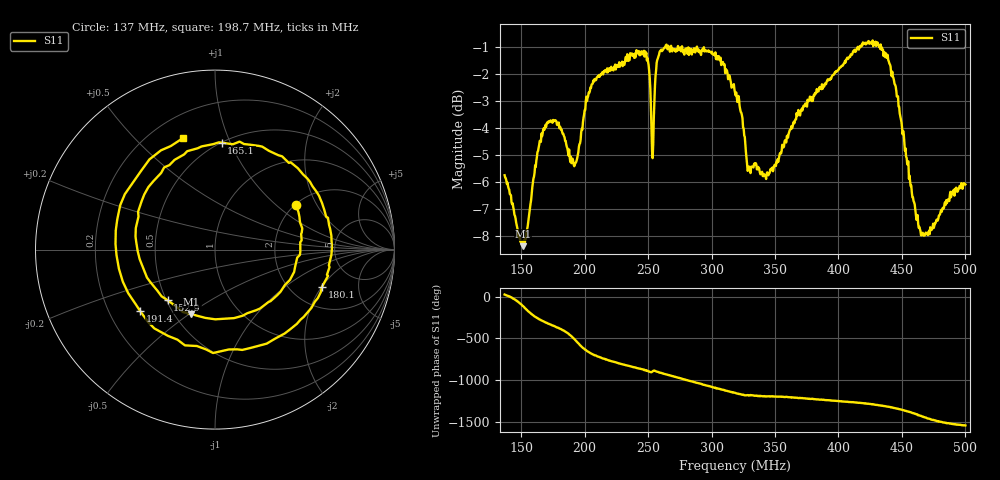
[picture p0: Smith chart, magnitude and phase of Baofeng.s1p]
#  HZ  S  RI  R  50.0
! Rohde & Schwarz ZVL
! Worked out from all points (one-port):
!   801 points, 137 MHz to 500 MHz, reference 50 ohm
!   lowest |S11| = -8.4 dB at 151.5 MHz (marker M1), VSWR 2.23, Z = 30.3 - j25.4 ohm
!   |S11| at or under -10 dB: nowhere
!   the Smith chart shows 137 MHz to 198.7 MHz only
!   S11 on the Smith chart (normalised r, x): 137 MHz: 2.03, +1.38; 152.9 MHz: 0.51, -0.34; 165.1 MHz: 0.50, +0.93; 180.1 MHz: 2.91, -2.01; 191.4 MHz: 0.33, -0.32; 198.7 MHz: 0.33, +0.70
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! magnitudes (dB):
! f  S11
! 137 MHz  -5.7
! 151.5 MHz  -8.4
! 152.9 MHz  -8.3
! 165.1 MHz  -4.5
! 171.9 MHz  -3.7
! 180.1 MHz  -4.0
! 182.4 MHz  -4.1
! 191.4 MHz  -5.4
! 198.7 MHz  -3.8
! 206.4 MHz  -2.3
! 227.8 MHz  -1.7
! 247.7 MHz  -1.2
! 250 MHz  -1.5
! 253.6 MHz  -5.1
! 258.6 MHz  -1.3
! 273.1 MHz  -1.1
! 301.3 MHz  -1.3
! 318.5 MHz  -2.7
! 329.8 MHz  -5.4
! 344.4 MHz  -5.7
! 363.9 MHz  -3.9
! 409.2 MHz  -1.4
! 425.1 MHz  -0.8
! 437.8 MHz  -1.3
! 445.1 MHz  -2.5
! 454.6 MHz  -5.3
! 466.4 MHz  -7.9
! 500 MHz  -6.1
